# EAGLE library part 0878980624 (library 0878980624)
CONN HEADER SMD 6POS 2.54MM Source: Datasheet
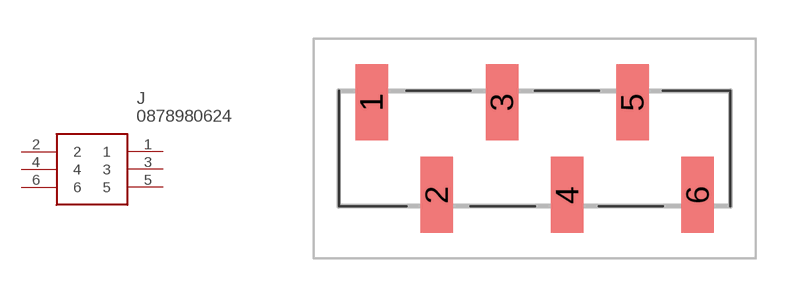
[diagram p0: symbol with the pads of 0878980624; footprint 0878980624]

Designator prefix J

## 0878980624 (Arrow_Part_Number: 0878980624; Arrow_Price-Stock: https://www.arrow.com/en/products/0878980624/molex; Description: CONN HEADER SMD 6POS 2.54MM; Height: 11.01mm; Manufacturer_Name: Molex; Manufacturer_Part_Number: 0878980624)  [0878980624]
1  1
2  2
3  3
4  4
5  5
6  6

## Footprint 0878980624 (pad centres in mm)
0878980624-2
smd 1.27 x 2.96: 1 -6.35,1.8; 2 -3.81,-1.8; 3 -1.27,1.8; 4 1.27,-1.8; 5 3.81,1.8; 6 6.35,-1.8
